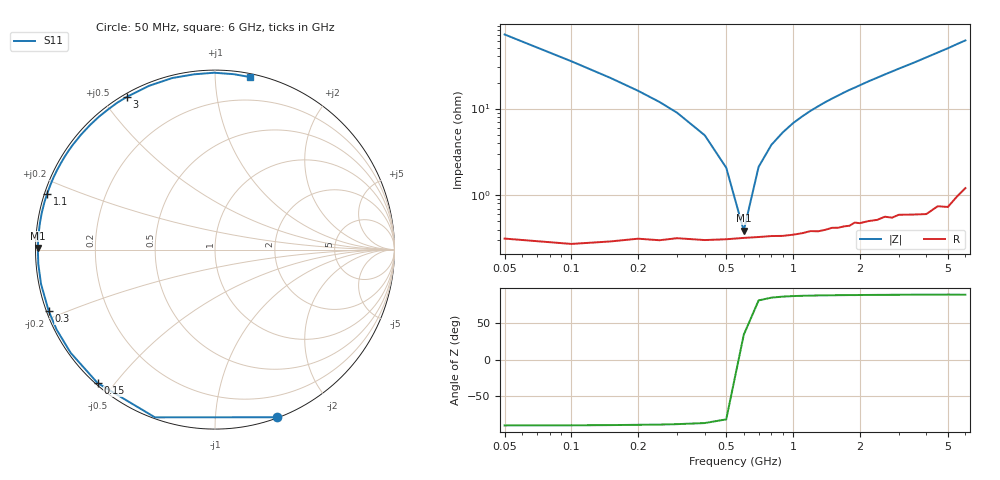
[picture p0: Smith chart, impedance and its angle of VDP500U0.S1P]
! Infineon Technologies  Discrete & RF Semiconductors
! BBY 55-03
! Si Tuning Diode in SOD323
! VR = 0.5 V
! S-Parameters:  June  1999
# GHz  S  MA  R  50
!  f  S11
! GHz  MAG  ANG
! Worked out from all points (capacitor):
!   34 points, 50 MHz to 6 GHz, reference 50 ohm
!   read as one part to ground: C = 43.9 pF near 50 MHz
!   lowest |Z| = 388 mohm at 600 MHz (marker M1)
!   series resonance near 590.4 MHz, so ESL is about 1.7 nH
!   S11 on the Smith chart (normalised r, x): 50 MHz: 0.01, -1.44; 150 MHz: 0.01, -0.45; 300 MHz: 0.01, -0.18; 1.1 GHz: 0.01, +0.16; 3 GHz: 0.01, +0.58; 6 GHz: 0.02, +1.23
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0.05  0.9959 -69.7
0.1  0.9927 -109.7
0.15  0.9904 -131.3
0.2  0.9887 -144.4
0.25  0.9887 -153.2
0.3  0.9878 -159.7
0.4  0.9881 -168.8
0.5  0.9877 -175.3
0.6  0.9873 179.5
0.7  0.987 175.2
0.8  0.9867 171.3
1  0.9864 164.6
1.1  0.986 161.6
1.2  0.9853 158.7
1.4  0.9851 153.3
1.6  0.9846 148.4
1.8  0.9841 143.6
2  0.9835 139.3
2.2  0.983 135.0
2.4  0.983 131.1
2.6  0.9821 127.2
3  0.9824 120.0
3.5  0.9838 111.9
4  0.9851 104.0
4.5  0.9835 96.8
5  0.9854 90.3
5.5  0.9829 83.9
6  0.9809 78.4
